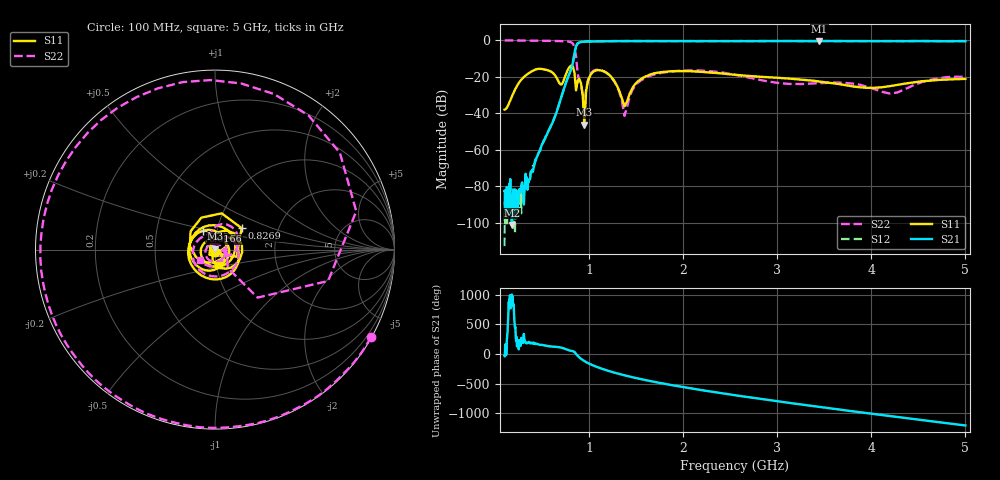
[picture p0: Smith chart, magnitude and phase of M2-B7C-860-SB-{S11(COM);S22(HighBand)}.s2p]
!Agilent Technologies,N5230A,MY45001737,A.07.50.48
!Agilent N5230A: A.07.50.48
!Date: Friday, August 11, 2023 17:40:05
!Correction: S11(Full 2 Port(1,4))
!S41(Full 2 Port(1,4))
!S14(Full 2 Port(1,4))
!S44(Full 2 Port(1,4))
!S2P File: Measurements: S11, S41, S14, S44:Log Frequency Sweep
# Hz S  MA  R 50
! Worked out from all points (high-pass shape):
!   201 points, 100 MHz to 5 GHz, reference 50 ohm
!   highest |S21| = -0.33 dB at 3.448 GHz (marker M1); lowest = -101.4 dB at 176.3 MHz (marker M2)
!   |S21| within 3 dB of the highest: 859.4 MHz to end of sweep
!   lowest |S11| = -46.2 dB at 948.2 MHz (marker M3), VSWR 1.01, Z = 49.8 + j0.462 ohm
!   |S11| at or under -10 dB: start of sweep to end of sweep
!   |S22| runs from -41.4 to 0.0 dB; largest |S21 - S12| = 0.016
!   S11 on the Smith chart (normalised r, x): 100 MHz: 0.99, -0.02; 616.6 MHz: 0.85, +0.18; 826.9 MHz: 1.30, +0.32; 5 GHz: 1.04, -0.18
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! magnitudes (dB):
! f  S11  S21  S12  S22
! 100 MHz  -38.0  -82.6  -113.0  0.0
! 176.3 MHz  -30.9  -101.4  -96.7  0.0
! 323.4 MHz  -19.3  -73.2  -80.8  -0.1
! 342.9 MHz  -18.5  -82.0  -77.3  -0.1
! 616.6 MHz  -18.0  -44.3  -44.1  -0.3
! 707.1 MHz  -24.1  -30.5  -30.4  -0.4
! 826.9 MHz  -14.4  -11.9  -11.9  -1.8
! 859.9 MHz  -27.4  -3.2  -3.2  -8.9
! 894.2 MHz  -21.1  -1.1  -1.1  -23.1
! 929.9 MHz  -29.4  -0.7  -0.7  -29.6
! 948.2 MHz  -46.2  -0.7  -0.6  -38.6
! 966.9 MHz  -27.5  -0.6  -0.6  -26.6
! 1.046 GHz  -17.1  -0.6  -0.6  -16.7
! 1.247 GHz  -20.9  -0.4  -0.4  -21.1
! 1.375 GHz  -36.1  -0.4  -0.3  -41.4
! 1.487 GHz  -24.1  -0.4  -0.3  -25.0
! 1.739 GHz  -17.6  -0.4  -0.4  -18.1
! 2.571 GHz  -19.0  -0.4  -0.3  -19.1
! 3.381 GHz  -22.1  -0.4  -0.3  -23.6
! 3.448 GHz  -22.6  -0.3  -0.3  -23.5
! 4.193 GHz  -25.1  -0.4  -0.3  -29.1
! 5 GHz  -21.1  -0.4  -0.4  -20.0
